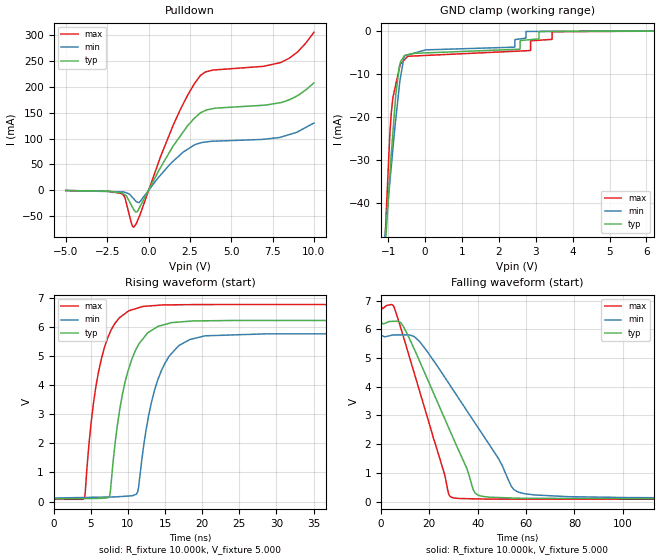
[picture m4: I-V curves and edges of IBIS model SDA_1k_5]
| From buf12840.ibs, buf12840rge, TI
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[Model] SDA_1k_5
|Signals SDA(15)
Model_type   I/O_open_drain
Polarity   Non-Inverting
Enable   Active-Low
Vinl = 1.5
Vinh = 3.5
Vmeas = 2.5
Vref = 2.5
Cref = 0pF
Rref = 10000
| Rpullup to DVDD = 1k
|   typ   min   max
|   (Nom PVT)   (Slow PVT)   (Fast PVT)
|  Output high impedance
|C_comp   2.0762000e-12  2.0690870e-12  2.1137920e-12
| Where   Nom PVT is  Nominal Process, 5.0V, 57C
|   Fast PVT is Strong Process, 5.5V, -40C
|   Slow PVT is Weak Process, 4.5V, 125C
|   typ   min   max
|   Output High
|   (Nom PVT)   (Slow PVT)   (Fast PVT)
C_comp   1.4979290e-10  1.0710390e-10  2.5469060e-10
| Where   Nom PVT is  Nominal Process, 5.0V, 57C
|   Fast PVT is Strong Process, 5.5V, -40C
|   Slow PVT is Weak Process, 4.5V, 125C
[Voltage Range]   5   4.5   5.5
[Temperature Range]   57   125   -40
|Ambient Temperature   27   95   -40
[Pullup Reference]   5   4.5   5.5
[Pulldown Reference]   -0   0   0
[Power Clamp Reference]   5   4.5   5.5
[GND Clamp Reference]   -0   0   -0
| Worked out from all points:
|   slope of the pulldown table from 0 to 0.75 V, typ, clamps not added: 16.5 ohm
|   falling waveform, R_fixture 10.000k, V_fixture 5.000: 20-80 % time 19.2ns typ, 26.2ns min, 14.2ns max; typ from 6.23 V to 0.09 V
|   rising waveform, R_fixture 10.000k, V_fixture 5.000: 20-80 % time 2.71ns typ, 2.98ns min, 2.44ns max; typ from 0.09 V to 6.23 V
[Pulldown]
|   Voltage   I(typ)   I(min)   I(max)
-5V       -663.8uA   -493.7uA   -664.8uA
-1.641V   -4.931mA   -3.205mA   -6.409mA
-1.43V    -9.095mA   -4.145mA   -14.81mA
-1.045V   -28.94mA   -11.56mA   -63.24mA
-897.8mV  -37.77mA   -16.77mA   -71.62mA
-539.1mV  -33.01mA   -22.85mA   -49.16mA
1.512V    86.91mA    56.92mA    127.7mA
3.12V     149.5mA    91.49mA    221.8mA
3.873V    157.9mA    94.91mA    232.8mA
7.98V     169.7mA    102.8mA    247.4mA
9.009V    183.4mA    113mA      268.1mA
10V       208mA      130.2mA    306mA
[GND Clamp]
|   Voltage   I(typ)   I(min)   I(max)
-5V       -625.4mA   -454.6mA   -1.011A
-1.074V   -49.05mA   -46.11mA   -46.07mA
-1.058V   -46.87mA   -44.57mA   -42.58mA
-960.4mV  -33.94mA   -35.39mA   -24.43mA
-883mV    -24.54mA   -28.1mA    -16.13mA
-697.4mV  -8.196mA   -12.57mA   -8.627mA
-558mV    -5.776mA   -5.903mA   -6.766mA
2.424V    -4.379mA   -3.857mA   -4.812mA
2.849V    -2.122mA   -215.3uA   -4.64mA
2.864V    -2.111mA   -214.9uA   -2.389mA
3.448V    -214.1uA   -197.2uA   -260.7uA
10V       0A         0A         0A
[POWER Clamp]
|   SCR cell for ESD function. Effects occurr above VDD x 2
|   Voltage   I(typ)   I(min)   I(max)
-5V       0A         0A         0A
0V        0A         0A         0A
10V       0A         0A         0A
[Ramp]
R_load = 10000
|   typ   min   max
dV/dt_r   2.94868/2.69641e-009   2.62912/2.96813e-009   3.26177/2.43922e-009
dV/dt_f   2.94868/1.92223e-008   2.62912/2.61958e-008   3.26177/1.42365e-008
[Falling Waveform]
R_fixture = 10.000k
V_fixture = 5.000
V_fixture_min = 4.500
V_fixture_max = 5.500
C_fixture = 0.000
|  time   V(typ)   V(min)   V(max)
0s        6.23V      5.771V     6.779V
5.647ns   6.282V     5.807V     6.733V
8.184ns   6.238V     5.806V     6.054V
13.83ns   5.302V     5.745V     4.458V
29.02ns   2.377V     3.995V     154.1mV
39.03ns   287.3mV    2.719V     92.95mV
48.59ns   138.9mV    1.501V     84.55mV
54.04ns   123.6mV    515.6mV    84.09mV
56.9ns    115.5mV    325.4mV    83.84mV
150ns     89.78mV    120.3mV    75.97mV
[Rising Waveform]
R_fixture = 10.000k
V_fixture = 5.000
V_fixture_min = 4.500
V_fixture_max = 5.500
C_fixture = 0.000
|  time   V(typ)   V(min)   V(max)
0s        89.78mV    120.3mV    75.97mV
4.172ns   102.3mV    140mV      117.7mV
5.691ns   106.9mV    147.2mV    3.941V
7.496ns   168.5mV    155.8mV    5.757V
9.262ns   3.679V     175.4mV    6.4V
11.32ns   5.343V     335mV      6.657V
11.91ns   5.559V     1.495V     6.704V
15.01ns   6.094V     4.769V     6.765V
20.46ns   6.218V     5.702V     6.777V
150ns     6.23V      5.771V     6.779V
